(* Logix 5000 AddOnInstructionDefinition export AKD_Home; software revision 26.01 *)

TYPE AKD_Status :   // All connections to the drive ethernet module are established and data is successfully transferring.
STRUCT
   Profile_In_Progress : BOOL;   // Profile Move In Progress
   Block_In_Execution : BOOL;   // Block In Execution
   On_Target_Position : BOOL;   // On Target Position (1=Current Position Equals Last Target Position)
   General_Fault : BOOL;   // General Fault
   Current_Direction : BOOL;   // Current Motor Direction (0=Reverse, 1=Forward)
   Home_Level : BOOL;   // Level of Home Input
   Reg_Level : BOOL;   // Level of Registration Input
   Enable : BOOL;   // State of Enable Output
   Fault_Input_Fault : BOOL;   // Fault Input Active
   Fwd_Limit : BOOL;   // Forward Input Active
   Rev_Limit : BOOL;   // Reverse Input Active
   Positive_Limit : BOOL;   // Positive Software Limit Exceeded
   Negative_Limit : BOOL;   // Negative Software Limit Exceeded
   FE_Fault : BOOL;   // Following Error Fault
   Block_Fault : BOOL;   // Block Execution Fault
   Load_Complete : BOOL;   // Command Message Successfully Loaded
END_STRUCT
END_TYPE

TYPE AKD_Control :   // Send Explicit Message
STRUCT
   Load_Data_Start_Profile : BOOL;   // Load Command Data / Start Profile Move
   Start_Block : BOOL;   // Execute Command block or block chain
   Incremental : BOOL;   // Incremental Position (0=Absolute, 1=Incremental)
   Direction : BOOL;   // Direction in Velocity Mode (0=Reverse, 1=Forward)
   Smooth_Stop : BOOL;   // Smooth / Controlled Stop w/ Deceleration
   Hard_Stop : BOOL;   // Hard / Immediate Stop
   Reg_Arm : BOOL;   // Arm the Registration Input
   Enable : BOOL;   // Enable Output
END_STRUCT
END_TYPE

TYPE AKD_Axis :   // Axis Data:
STRUCT
   Control : AKD_Control;   // Control bits to send to the drive
   Status : AKD_Status;   // Status bits received from the drive
   Input : AB:ETHERNET_MODULE_SINT_64Bytes:I:0;   // Data from the drive
   Output : AB:ETHERNET_MODULE_SINT_64Bytes:O:0;   // Data to the drive
   ResponseMsgType : SINT;   // Response type contained in latest IO response from drive. Used to check for errors
   CommandTimeout : INT;   // Time to allow for command response from drive. Dependent on scan rate and communicaiton rate
   PositionFeedback : DINT;   // Actual Position Value
   VelocityFeedback : DINT;   // Actual Velocity Value
END_STRUCT
END_TYPE

ADD_ON_INSTRUCTION AKD_Set_Attribute   (* revision 2.1, ExecutePrescan, ExecuteEnableInFalse *)
// Set Position Controller Attribute
// Revision note:
// Don't error if Command_Timeout preset is 0
VAR_OUTPUT
   DN : BOOL; {access Read Only, visible}   // Command Successful
   ER : BOOL; {access Read Only, visible}   // Error
END_VAR
VAR_IN_OUT
   Axis : AKD_Axis; {required}
END_VAR
VAR_INPUT
   Attribute_Number : INT; {visible}   // Attribute Number (see help for options)
   Attribute_Value : DINT; {required}   // Attribute Value
END_VAR
VAR
   Command_Timeout : TIMER := (PRE := 200);   // Timeout Timer
   Command_Message_Type : SINT;   // Command Message Type
   Command_Axis_Number : SINT;   // Command Axis Number
   Step : SINT;
   Command_Bytes : SINT[8];
   OS_LoadStart : BOOL;
END_VAR

ROUTINE EnableInFalse   (* ladder *)
// EnableIn_False
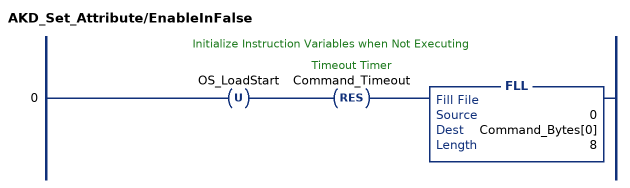
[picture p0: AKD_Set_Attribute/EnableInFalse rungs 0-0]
   // Initialize Instruction Variables when Not Executing
   0: OTU(OS_LoadStart)RES(Command_Timeout)FLL(0,Command_Bytes[0],8);
END_ROUTINE

ROUTINE Logic   (* ladder *)
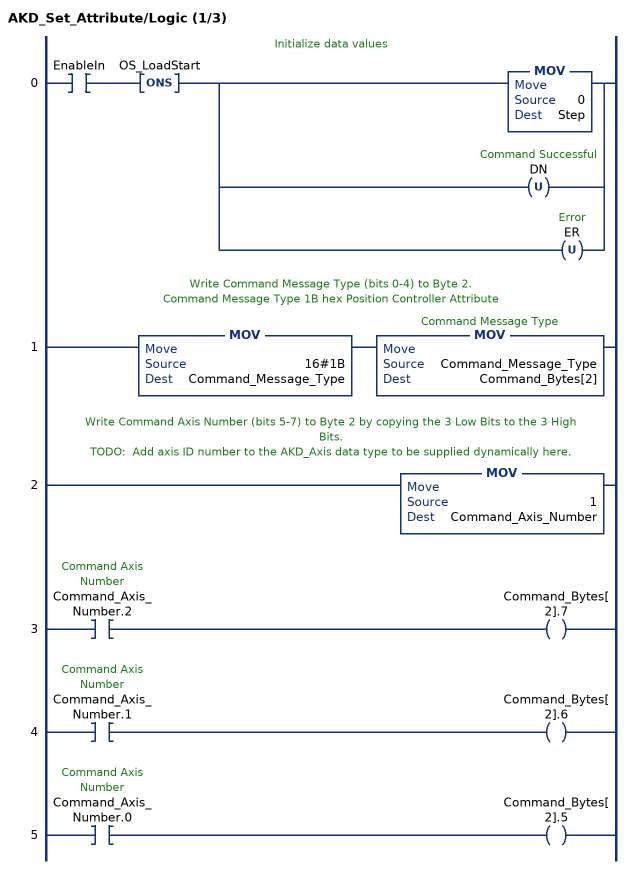
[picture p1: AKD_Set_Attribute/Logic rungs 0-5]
   // Initialize data values
   0: XIC(EnableIn)ONS(OS_LoadStart)[MOV(0,Step) ,OTU(DN) ,OTU(ER) ];
   // Write Command Message Type (bits 0-4) to Byte 2.
   // Command Message Type 1B hex Position Controller Attribute
   1: MOV(16#1B,Command_Message_Type)MOV(Command_Message_Type,Command_Bytes[2]);
   // Write Command Axis Number (bits 5-7) to Byte 2 by copying the 3 Low Bits to the 3 High Bits.
   // TODO:  Add axis ID number to the AKD_Axis data type to be supplied dynamically here.
   2: MOV(1,Command_Axis_Number);
   3: XIC(Command_Axis_Number.2)OTE(Command_Bytes[2].7);
   4: XIC(Command_Axis_Number.1)OTE(Command_Bytes[2].6);
   5: XIC(Command_Axis_Number.0)OTE(Command_Bytes[2].5);
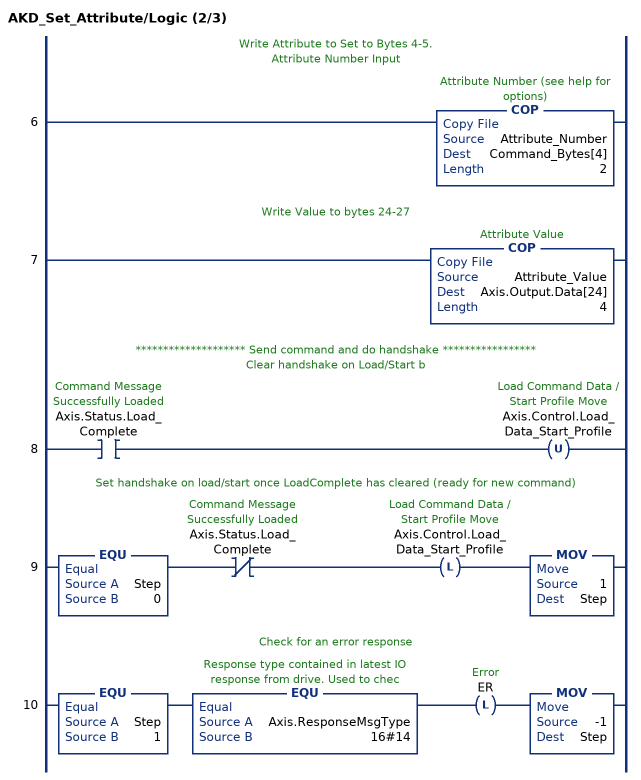
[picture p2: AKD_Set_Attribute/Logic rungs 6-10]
   // Write Attribute to Set to Bytes 4-5.
   // Attribute Number Input
   6: COP(Attribute_Number,Command_Bytes[4],2);
   // Write Value to bytes 24-27
   7: COP(Attribute_Value,Axis.Output.Data[24],4);
   // ******************** Send command and do handshake *****************
   // Clear handshake on Load/Start b
   8: XIC(Axis.Status.Load_Complete)OTU(Axis.Control.Load_Data_Start_Profile);
   // Set handshake on load/start once LoadComplete has cleared (ready for new command)
   9: EQU(Step,0)XIO(Axis.Status.Load_Complete)OTL(Axis.Control.Load_Data_Start_Profile)MOV(1,Step);
   // Check for an error response
   10: EQU(Step,1)EQU(Axis.ResponseMsgType,16#14)OTL(ER)MOV(-1,Step);
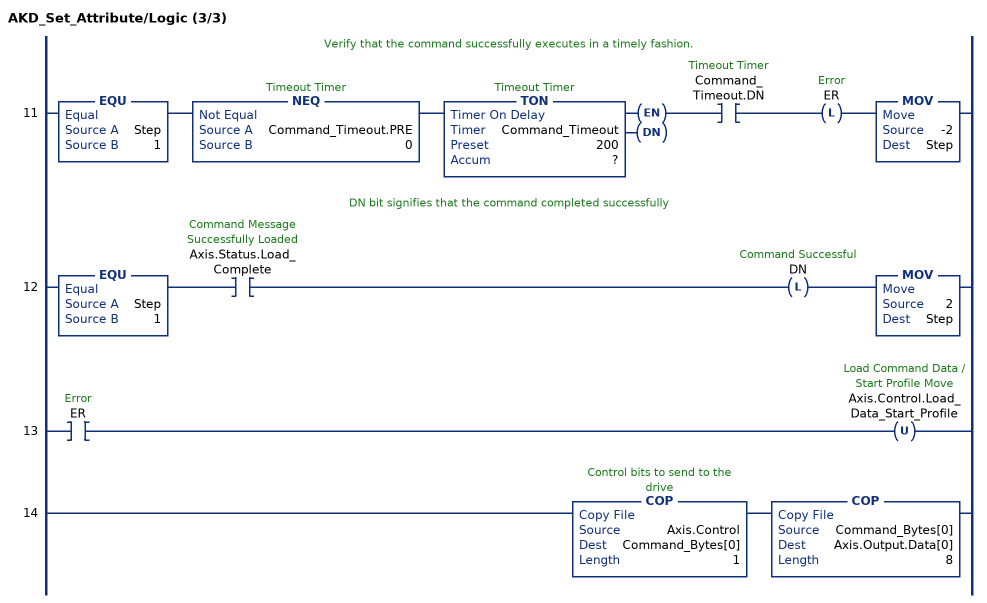
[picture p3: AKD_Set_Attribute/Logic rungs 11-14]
   // Verify that the command successfully executes in a timely fashion.
   11: EQU(Step,1)NEQ(Command_Timeout.PRE,0)TON(Command_Timeout,?,?)XIC(Command_Timeout.DN)OTL(ER)MOV(-2,Step);
   // DN bit signifies that the command completed successfully
   12: EQU(Step,1)XIC(Axis.Status.Load_Complete)OTL(DN)MOV(2,Step);
   13: XIC(ER)OTU(Axis.Control.Load_Data_Start_Profile);
   14: COP(Axis.Control,Command_Bytes[0],1)COP(Command_Bytes[0],Axis.Output.Data[0],8);
END_ROUTINE

ROUTINE Prescan   (* ladder *)
// Prescan
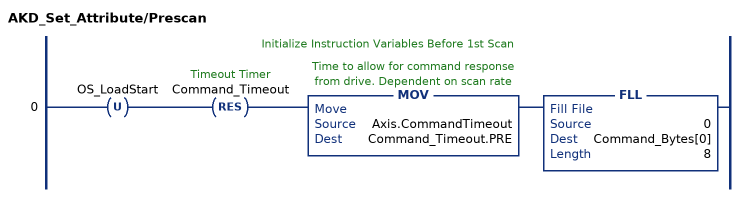
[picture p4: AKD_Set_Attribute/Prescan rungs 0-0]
   // Initialize Instruction Variables Before 1st Scan
   0: OTU(OS_LoadStart)RES(Command_Timeout)MOV(Axis.CommandTimeout,Command_Timeout.PRE)FLL(0,Command_Bytes[0],8);
END_ROUTINE
END_ADD_ON_INSTRUCTION

ADD_ON_INSTRUCTION AKD_Home   (* revision 4.0, ExecutePrescan, ExecuteEnableInFalse *)
// Home Axis
// Revision note:
// added timeout
// removed race with SetAttribute.dn bit
VAR_OUTPUT
   DN : BOOL; {access Read Only, visible}   // Command Successfully Initiated
   ER : BOOL; {access Read Only, visible}   // Error
   IP : BOOL; {access Read Only, visible}   // Command in Process
   PC : BOOL; {access Read Only, visible}   // Command Process Complete
END_VAR
VAR_IN_OUT
   Axis : AKD_Axis; {required}
END_VAR
VAR_INPUT
   TimeOut_mS : DINT; {required}
END_VAR
VAR
   Step : SINT;
   Set_Attribute : AKD_Set_Attribute;
   Value : DINT;
   StartONS : BOOL;
   TimeOut : TIMER := (PRE := 5000); {access None}
END_VAR

ROUTINE EnableInFalse   (* ladder *)
// EnableIn_False
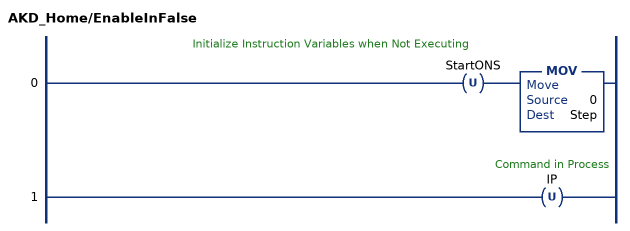
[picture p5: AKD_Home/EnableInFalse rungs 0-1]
   // Initialize Instruction Variables when Not Executing
   0: OTU(StartONS)MOV(0,Step);
   1: OTU(IP);
END_ROUTINE

ROUTINE Logic   (* ladder *)
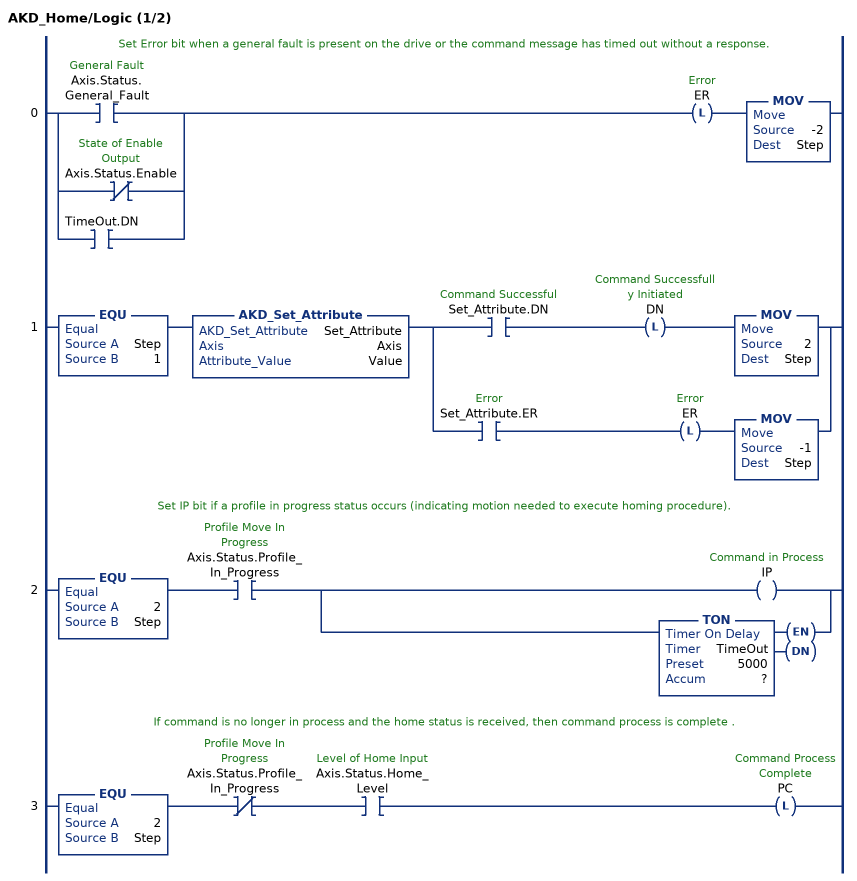
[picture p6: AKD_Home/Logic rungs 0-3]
   // Set Error bit when a general fault is present on the drive or the command message has timed out without a response.
   0: [XIC(Axis.Status.General_Fault) ,XIO(Axis.Status.Enable) ,XIC(TimeOut.DN) ]OTL(ER)MOV(-2,Step);
   1: EQU(Step,1)AKD_Set_Attribute(Set_Attribute,Axis,Value)[XIC(Set_Attribute.DN) OTL(DN) MOV(2,Step) ,XIC(Set_Attribute.ER) OTL(ER) MOV(-1,Step) ];
   // Set IP bit if a profile in progress status occurs (indicating motion needed to execute homing procedure).
   2: EQU(2,Step)XIC(Axis.Status.Profile_In_Progress)[OTE(IP) ,TON(TimeOut,?,?) ];
   // If command is no longer in process and the home status is received, then command process is complete .
   3: EQU(2,Step)XIO(Axis.Status.Profile_In_Progress)XIC(Axis.Status.Home_Level)OTL(PC);
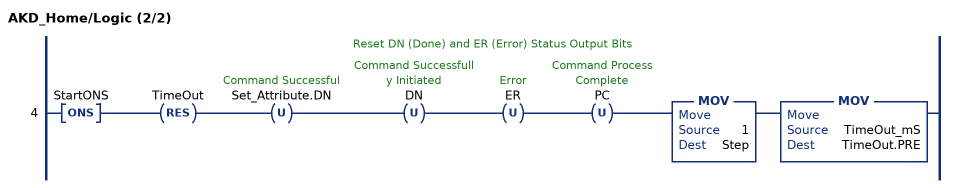
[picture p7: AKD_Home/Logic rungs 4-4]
   // Reset DN (Done) and ER (Error) Status Output Bits
   4: ONS(StartONS)RES(TimeOut)OTU(Set_Attribute.DN)OTU(DN)OTU(ER)OTU(PC)MOV(1,Step)MOV(TimeOut_mS,TimeOut.PRE);
END_ROUTINE

ROUTINE Prescan   (* ladder *)
// Prescan
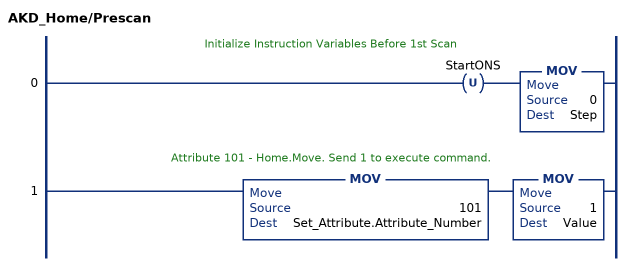
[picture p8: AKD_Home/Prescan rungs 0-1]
   // Initialize Instruction Variables Before 1st Scan
   0: OTU(StartONS)MOV(0,Step);
   // Attribute 101 - Home.Move. Send 1 to execute command.
   1: MOV(101,Set_Attribute.Attribute_Number)MOV(1,Value);
END_ROUTINE
END_ADD_ON_INSTRUCTION
